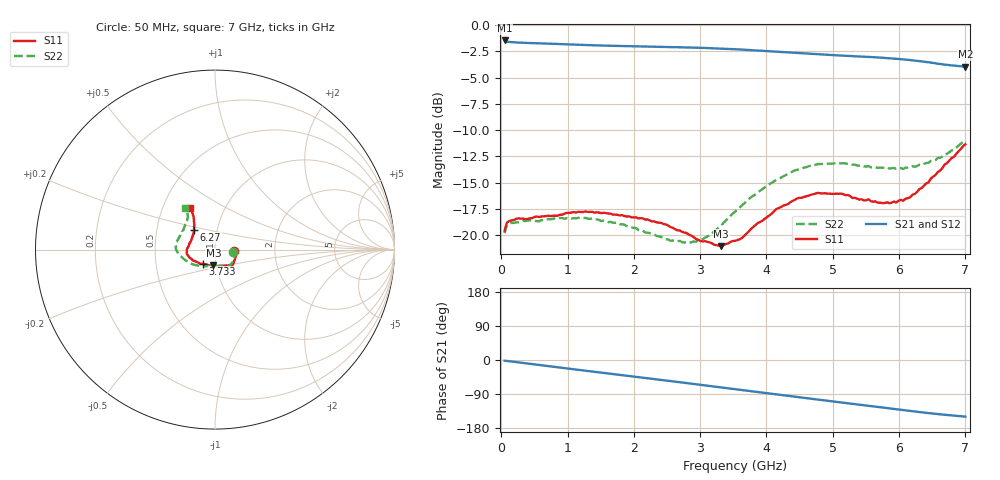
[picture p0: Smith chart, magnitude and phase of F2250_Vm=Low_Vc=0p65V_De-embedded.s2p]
! Integrated Device Technology
! Corporate Headquarters
! 6024 Silver Creek Valley Road
! San Jose, CA 95138  USA
! Phone:  1-408-284-8200
! Toll Free:  1-800-223-1366
! Webpage:  http://www.idt.com/
! Timing and RF Division
! 515 Groton Road, Suite 102
! Westford, MA 01886-6024
! Device:  F2250
! Description: Voltage Variable RF Attenuator
! Frequency:  50.0 -  6000.00 MHz
! Package:  3x3 mm Thin QFN Plastic Package: 16 pin
! Ports:  2 RF, 3 DC
!  Pin  1  = GND
!  Pin  2  = NC
!  Pin  3  = RF1  = Port 1
!  Pin  4  = NC
!  Pin  5  = GND
!  Pin  6  = GND
!  Pin  7  = GND
!  Pin  8  = GND
!  Pin  9  = NC
!  Pin 10  = RF2  = Port 2
!  Pin 11  = NC
!  Pin 12  = GND
!  Pin 13  = GND
!  Pin 14  = VCNTRL
!  Pin 15  = VDD
!  Pin 16  = VMODE
! Vcntrl:  0.650 Volts
! Vmode:  +0.000 Volts
! Vdd:  +3.30  Volts
! Current:  1.144 mA
! Data:  The device was measured on a the F2250 evaluation board which has
!  individual transmission lines to the RF pins.  Data was collected
!  using a calibrated network analyzer.  The evaluation board was
!  de-embedded using a TRL calibration technique.
!  The reference plane is the edge of the package pin.
! Misc:  SN 10
!  Action Tracker AT0258
! Date Measured:  2014-11-26
! Date:  2015-10-15  MJV
! Note:
!  Integrated Device Technology supplies this data as a sample of measured
!  data at the package pin for this product.  Your particular data for this
!  product may vary.
!  Data was taken at 25 degrees C.
!  Integrated Device Technology reserves the right to change this data at anytime.
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# GHz S dB R 50
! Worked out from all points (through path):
!   201 points, 50 MHz to 7 GHz, reference 50 ohm
!   highest |S21| = -1.45 dB at 50 MHz (marker M1); lowest = -4.0 dB at 7 GHz (marker M2)
!   group delay of S21, straight-line fit = 60 ps
!   lowest |S11| = -21.1 dB at 3.317 GHz (marker M3), VSWR 1.19, Z = 48.3 - j8.59 ohm
!   |S11| at or under -10 dB: start of sweep to end of sweep
!   |S22| runs from -20.7 to -10.9 dB; largest |S21 - S12| = 0.00062
!   S11 on the Smith chart (normalised r, x): 50 MHz: 1.23, -0.02; 3.733 GHz: 0.86, -0.14; 6.27 GHz: 0.77, +0.18; 7 GHz: 0.69, +0.35
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0.05  -19.56 -5.0  -1.45 -1.9  -1.45 -1.8  -19.81 -6.4
0.08475  -18.81 -5.3  -1.56 -2.5  -1.56 -2.5  -19.02 -6.3
0.22375  -18.45 -9.5  -1.65 -5.5  -1.64 -5.5  -18.79 -11.2
0.71025  -18.15 -26.2  -1.76 -16.2  -1.76 -16.2  -18.46 -31.2
1.2315  -17.80 -40.5  -1.88 -27.5  -1.88 -27.5  -18.38 -50.3
1.75275  -18.06 -47.3  -1.98 -38.5  -1.98 -38.5  -18.81 -61.1
2.37825  -18.82 -51.0  -2.06 -51.8  -2.06 -51.8  -20.12 -72.0
2.552  -19.23 -53.9  -2.09 -55.5  -2.08 -55.5  -20.55 -77.9
2.93425  -20.35 -67.3  -2.14 -64.0  -2.15 -64.0  -20.63 -98.3
3.14275  -20.69 -81.2  -2.18 -68.6  -2.18 -68.6  -20.03 -113.4
3.3165  -21.05 -95.9  -2.23 -72.5  -2.22 -72.5  -19.08 -124.5
3.525  -20.54 -113.4  -2.29 -77.1  -2.29 -77.1  -17.78 -136.5
3.7335  -19.64 -130.3  -2.36 -81.8  -2.36 -81.8  -16.58 -146.5
4.1505  -17.51 -151.9  -2.53 -91.0  -2.53 -91.0  -14.73 -164.1
4.7065  -16.10 -170.0  -2.74 -103.0  -2.74 -103.0  -13.36 -179.1
5.1235  -16.04 179.9  -2.89 -112.0  -2.89 -112.0  -13.16 171.6
5.471  -16.70 168.9  -3.00 -119.4  -3.00 -119.4  -13.45 164.2
5.85325  -16.96 154.9  -3.15 -127.5  -3.16 -127.6  -13.65 154.5
6.06175  -16.72 145.9  -3.25 -132.1  -3.26 -132.1  -13.70 148.4
6.27025  -15.88 136.6  -3.39 -136.6  -3.39 -136.6  -13.42 141.8
6.61775  -13.86 124.8  -3.69 -143.3  -3.69 -143.3  -12.63 130.1
7  -11.33 120.4  -3.96 -149.5  -3.96 -149.5  -10.94 125.6
